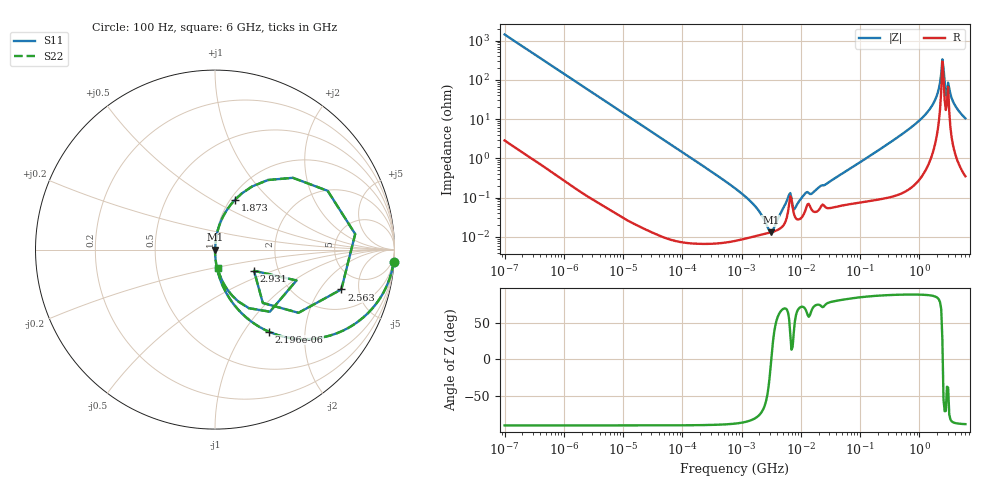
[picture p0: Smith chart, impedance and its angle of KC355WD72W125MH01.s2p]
!Murata Part Number: KC355WD72W125MH01
!These Parameters are Measured in Series Mode Connection
!Data Generated on Jun 19, 2026
!  o--ll--o
!Port1  Port2
!  o------o
!Operation Temp=25[degC], DC Bias Voltage=0[V]
!Freq. Start=100[Hz] Stop=6[GHz] 401[Steps]
# Hz S RI R 50
!Freq.(Hz) S11(Real) S11(Imag) S21(Real) S21(Imag) S12(Real) S12(Imag) S22(Real) S22(Imag)
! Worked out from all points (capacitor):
!   401 points, 100 Hz to 6 GHz, reference 50 ohm
!   read as one part in series: C = 1.11 uF near 109 Hz
!   lowest |Z| = 13.2 mohm at 3.104 MHz (marker M1)
!   series resonance near 3.172 MHz, so ESL is about 2.3 nH
!   S11 on the Smith chart (normalised r, x): 100 Hz: 1, -29; 2.196 kHz: 1.00, -1.31; 1.873 GHz: 1.05, +0.64; 2.563 GHz: 3.33, -3.24; 2.931 GHz: 1.50, -0.38; 6 GHz: 1.01, -0.21
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100  0.995 -0.0696  0.005 0.0696  0.005 0.0696  0.995 -0.0696
548  0.8719 -0.3333  0.1281 0.3333  0.1281 0.3333  0.8719 -0.3333
2008  0.3384 -0.4722  0.6616 0.4722  0.6616 0.4722  0.3384 -0.4722
2196  0.2996 -0.4572  0.7004 0.4572  0.7004 0.4572  0.2996 -0.4572
6151  0.0522 -0.2213  0.9478 0.2213  0.9478 0.2213  0.0522 -0.2213
40335  0.00138 -0.0356  0.9986 0.0356  0.9986 0.0356  0.00138 -0.0356
774597  8.2e-05 -0.00173  0.9999 0.00173  0.9999 0.00173  8.2e-05 -0.00173
1734173  0.000105 -0.000572  0.9999 0.000572  0.9999 0.000572  0.000105 -0.000572
3103719  0.00013 -1.97e-05  0.9999 1.97e-05  0.9999 1.97e-05  0.00013 -1.97e-05
3549919  0.000139 0.000105  0.9999 -0.000105  0.9999 -0.000105  0.000139 0.000105
6075234  0.000433 0.00089  0.9996 -0.00089  0.9996 -0.00089  0.000433 0.00089
7947587  0.000327 0.00042  0.9997 -0.00042  0.9997 -0.00042  0.000327 0.00042
1.189169e7  0.000468 0.0012  0.9995 -0.0012  0.9995 -0.0012  0.000468 0.0012
1.555665e7  0.000474 0.0012  0.9995 -0.0012  0.9995 -0.0012  0.000474 0.0012
3.124326e8  0.00162 0.0246  0.9984 -0.0246  0.9984 -0.0246  0.00162 0.0246
1.046602e9  0.0125 0.0962  0.9875 -0.0962  0.9875 -0.0962  0.0125 0.0962
1.873145e9  0.1124 0.2788  0.8876 -0.2788  0.8876 -0.2788  0.1124 0.2788
2.240541e9  0.4339 0.4  0.5661 -0.4  0.5661 -0.4  0.4339 0.4
2.562649e9  0.7039 -0.2218  0.2961 0.2218  0.2961 0.2218  0.7039 -0.2218
2.931063e9  0.2174 -0.1179  0.7826 0.1179  0.7826 0.1179  0.2174 -0.1179
3.8344e9  0.074 -0.2297  0.926 0.2297  0.926 0.2297  0.074 -0.2297
6e9  0.0142 -0.1027  0.9858 0.1027  0.9858 0.1027  0.0142 -0.1027
